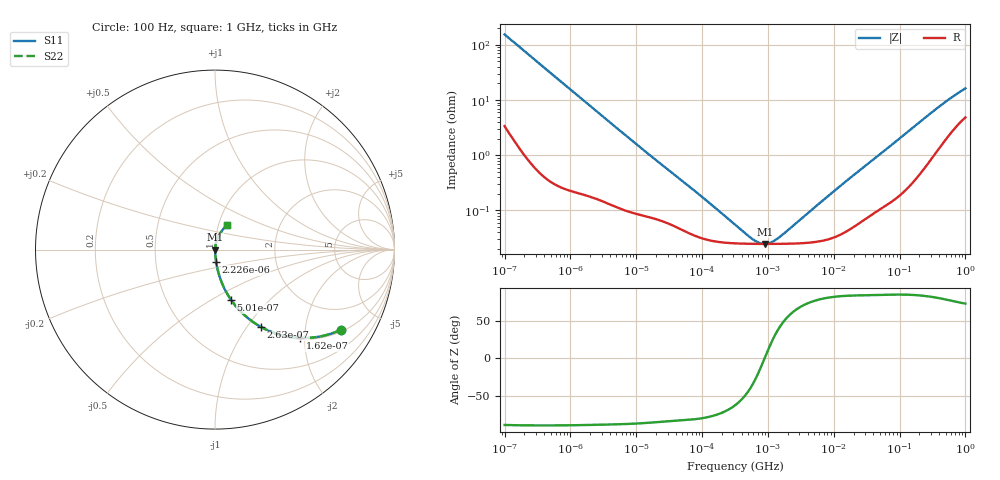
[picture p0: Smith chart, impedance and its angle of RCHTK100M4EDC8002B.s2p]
! RCHTK100M4EDC8002B  S-PARAMETER MODEL  (AEC-Q200 qualified)
! Model Generated by ELNA Corporation (http://www.ty-top.com)
! Version 1.0
! ELNA Control No. 240315
! Copyright (c) 2024 ELNA CO.,LTD. All Rights Reserved.
! Products Name : CONDUCTIVE POLYMER HYBRID ALUMINUM ELECTROLYTIC CAPACITORS
! Characteristics :
!  Capacitance  :  10uF  ,  Rated voltage  :  63V
!  Operating Temp. Range  :  -55 to +125 degC  ,  Endurance  :  6000hr at 125 degC
!  Dimension D  :  6.3mm  ,  Dimension L  :  5.8mm
! Frequency Range : 100Hz - 1GHz
! External Node Assignments :
!  1  o---| |---o  2
# MHz S RI R 50
!Freq[MHz].  S11 Real  S11 Imag  S21 Real  S21 Imag  S12 Real  S12 Imag  S22 Real  S22 Imag
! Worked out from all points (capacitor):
!   401 points, 100 Hz to 1 GHz, reference 50 ohm
!   read as one part in series: C = 10.3 uF near 108 Hz
!   lowest |Z| = 24.8 mohm at 901.6 kHz (marker M1)
!   series resonance near 892.2 kHz, so ESL is about 3.1 nH
!   S11 on the Smith chart (normalised r, x): 100 Hz: 1.07, -3.08; 162 Hz: 1.03, -1.90; 263 Hz: 1.01, -1.17; 501 Hz: 1.01, -0.62; 2.226 kHz: 1.00, -0.14; 1 GHz: 1.10, +0.31
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0.0001  0.6994 -0.4477  0.3006 0.4477  0.3006 0.4477  0.6994 -0.4477
0.000162  0.4746 -0.492  0.5254 0.492  0.5254 0.492  0.4746 -0.492
0.000263  0.2578 -0.4318  0.7422 0.4318  0.7422 0.4318  0.2578 -0.4318
0.000363  0.1552 -0.3569  0.8448 0.3569  0.8448 0.3569  0.1552 -0.3569
0.000501  0.0889 -0.2793  0.9111 0.2793  0.9111 0.2793  0.0889 -0.2793
0.000846  0.0344 -0.1757  0.9656 0.1757  0.9656 0.1757  0.0344 -0.1757
0.001488  0.0126 -0.1025  0.9874 0.1025  0.9874 0.1025  0.0126 -0.1025
0.002226  0.00652 -0.0693  0.9935 0.0693  0.9935 0.0693  0.00652 -0.0693
0.005623  0.00187 -0.0279  0.9981 0.0279  0.9981 0.0279  0.00187 -0.0279
0.022131  0.000725 -0.00736  0.9993 0.00736  0.9993 0.00736  0.000725 -0.00736
0.087096  0.000335 -0.00199  0.9997 0.00199  0.9997 0.00199  0.000335 -0.00199
0.316228  0.000254 -0.000491  0.9997 0.000491  0.9997 0.000491  0.000254 -0.000491
0.627336  0.000249 -0.000143  0.9998 0.000143  0.9998 0.000143  0.000249 -0.000143
0.767361  0.000248 -6.03e-05  0.9998 6.03e-05  0.9998 6.03e-05  0.000248 -6.03e-05
0.901571  0.000248 4.21e-06  0.9998 -4.21e-06  0.9998 -4.21e-06  0.000248 4.21e-06
1.102808  0.000248 8.52e-05  0.9998 -8.52e-05  0.9998 -8.52e-05  0.000248 8.52e-05
1.40443  0.000248 0.000187  0.9998 -0.000187  0.9998 -0.000187  0.000248 0.000187
4.704354  0.000266 0.00101  0.9997 -0.00101  0.9997 -0.00101  0.000266 0.00101
69.9842  0.00155 0.0142  0.9985 -0.0142  0.9985 -0.0142  0.00155 0.0142
395.8221  0.0183 0.0721  0.9817 -0.0721  0.9817 -0.0721  0.0183 0.0721
668.3439  0.0406 0.1077  0.9594 -0.1077  0.9594 -0.1077  0.0406 0.1077
1000  0.0667 0.1383  0.9333 -0.1383  0.9333 -0.1383  0.0667 0.1383
